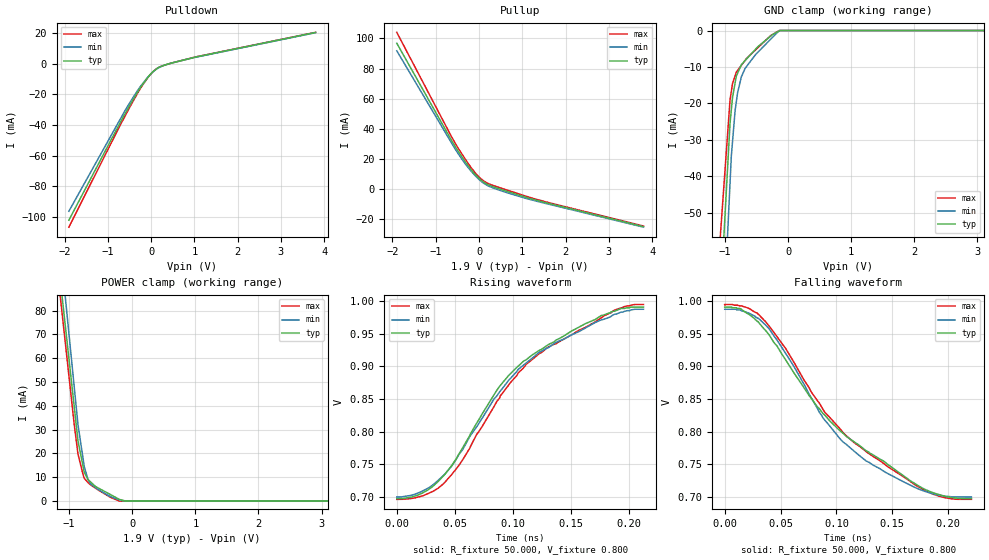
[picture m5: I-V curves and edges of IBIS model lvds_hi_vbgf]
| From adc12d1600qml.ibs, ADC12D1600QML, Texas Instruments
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[Model]   lvds_hi_vbgf
Model_type Output
Vref=0.80E+00
Rref=5.000E+01
Cref=0.000E+00
Vmeas=0.80E+00
C_comp   4.84E-13   4.84E-13   4.84E-13
[Voltage Range]   1.900E+00   1.800E+00   2.000E+00
[POWER Clamp Reference]   1.900E+00   1.800E+00   2.000E+00
[GND Clamp Reference]   0.000E+00   0.000E+00   0.000E+00
[Pullup Reference]   1.900E+00   1.800E+00   2.000E+00
[Pulldown Reference]   0.000E+00   0.000E+00   0.000E+00
[Temperature Range]   25   85   -40
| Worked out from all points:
|   slope of the pulldown table from 0 to 0.285 V, typ, clamps not added: 53.7 ohm
|   slope of the pullup table from 0 to 0.285 V, typ, clamps not added: 56 ohm
|   GND clamp passes 1 mA (typ) near -0.24 V on its own axis
|   POWER clamp passes 1 mA (typ) near -0.22 V on its own axis
|   rising waveform, R_fixture 50.000, V_fixture 0.800: 20-80 % time 79.3ps typ, 80.7ps min, 81.3ps max; typ from 0.697 V to 0.991 V
|   falling waveform, R_fixture 50.000, V_fixture 0.800: 20-80 % time 94.7ps typ, 74.1ps min, 87.2ps max; typ from 0.991 V to 0.697 V
[GND Clamp]
-2V       -368.8mA   -437.3mA   -281.6mA
-1.8V     -305.2mA   -364mA     -232.9mA
-920mV    -25.41mA   -41.86mA   -19.01mA
-900mV    -21.84mA   -34.54mA   -16.75mA
-880mV    -18.27mA   -30.36mA   -14.49mA
-840mV    -14.43mA   -21.99mA   -12.43mA
-800mV    -11.72mA   -17.02mA   -10.94mA
-740mV    -9.361mA   -12.67mA   -9.542mA
-680mV    -8.227mA   -10.36mA   -8.148mA
-520mV    -5.203mA   -6.699mA   -5.383mA
-140mV    -173.1uA   0A         0A
4V        0A         0A         0A
[POWER Clamp]
-2.1V     323.5mA    363.2mA    318.9mA
-1.7V     227.3mA    255.8mA    221.7mA
-980mV    54.15mA    64.06mA    46.82mA
-920mV    39.72mA    48.08mA    32.25mA
-860mV    25.29mA    32.1mA     19.78mA
-760mV    12.02mA    14.43mA    9.543mA
-700mV    9.016mA    8.989mA    7.766mA
-660mV    8.043mA    7.222mA    6.814mA
-360mV    2.964mA    2.076mA    1.818mA
-200mV    684.4uA    475.1uA    0A
-100mV    0A         0A         0A
3.9V      0A         0A         0A
[Pullup]
-1.9V     96.8mA     91.77mA    104mA
-540mV    27.86mA    26.16mA    29.98mA
-340mV    19.09mA    17.71mA    20.93mA
-180mV    12.8mA     11.9mA     14.21mA
-60mV     8.879mA    8.13mA     9.93mA
100mV     4.778mA    4.124mA    5.661mA
200mV     3.101mA    2.368mA    3.946mA
400mV     916uA      60.01uA    1.759mA
1.08V     -5.366mA   -6.072mA   -4.6mA
1.74V     -10.33mA   -10.83mA   -9.824mA
3.8V      -24.81mA   -25.16mA   -24.42mA
[Pulldown]
-1.9V     -102.1mA   -96.29mA   -106.6mA
-700mV    -37.62mA   -35.47mA   -39.3mA
-460mV    -25.49mA   -23.94mA   -26.65mA
-240mV    -15.29mA   -14.58mA   -15.8mA
-100mV    -9.804mA   -9.572mA   -9.977mA
0V        -6.456mA   -6.47mA    -6.458mA
100mV     -3.853mA   -3.979mA   -3.792mA
320mV     -807.4uA   -839.7uA   -818.3uA
1V        4.194mA    4.063mA    4.265mA
3.8V      20.43mA    20.28mA    20.51mA
[Rising Waveform]
R_fixture = 50.000
V_fixture = 0.800
V_fixture_min = 0.800
V_fixture_max = 0.800
|  time   V(typ)   V(min)   V(max)
0s        697.1mV    699.7mV    696.1mV
22.25ps   705.9mV    708.9mV    701.4mV
40.5ps    732.5mV    733.1mV    720.4mV
56.75ps   774.9mV    772.2mV    756.5mV
88.75ps   869.7mV    861.1mV    851.7mV
109.2ps   908mV      901.9mV    897.7mV
130.7ps   933.5mV    928.7mV    929.7mV
176.5ps   978.2mV    971.6mV    974.6mV
196.2ps   988.9mV    984.4mV    991.8mV
212.7ps   991mV      987.7mV    995mV
[Falling Waveform]
R_fixture = 50.000
V_fixture = 0.800
V_fixture_min = 0.800
V_fixture_max = 0.800
|  time   V(typ)   V(min)   V(max)
0s        991mV      987.7mV    995mV
14.75ps   987.8mV    985.5mV    992.8mV
28.75ps   969.7mV    974.8mV    982.1mV
39.75ps   948.4mV    957.6mV    961.8mV
62ps      889.9mV    899.7mV    906.2mV
87.75ps   828.1mV    821.5mV    834.6mV
106ps     797.3mV    783.9mV    798.2mV
126.5ps   770.7mV    755mV      769.4mV
181.5ps   709.6mV    707.1mV    707.6mV
220.7ps   697.1mV    699.7mV    696.1mV
[Ramp]
dV/dt_r   1.7621E+00/7.9160E-11   1.7024E+00/8.0480E-11   1.8222E+00/8.0750E-11
dV/dt_f   1.7621E+00/9.4438E-11   1.7024E+00/7.4086E-11   1.8222E+00/8.6703E-11
R_load = 50
